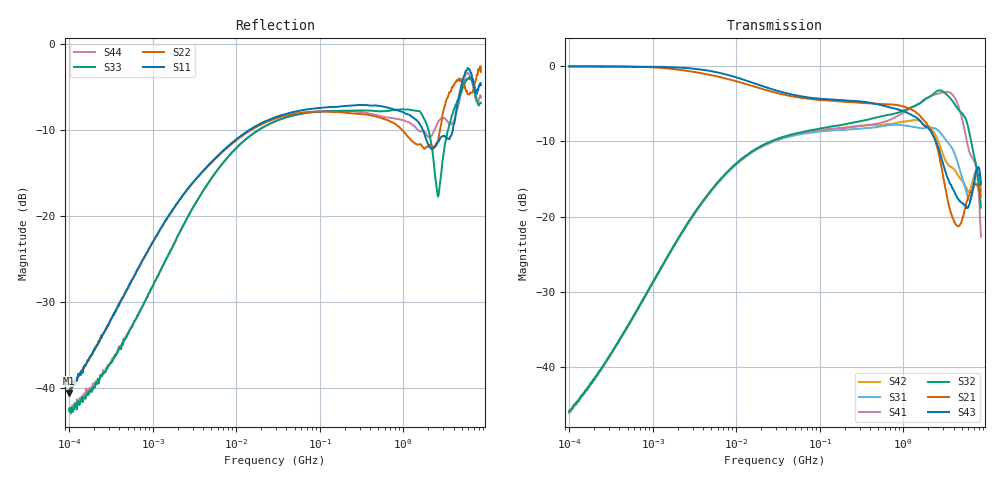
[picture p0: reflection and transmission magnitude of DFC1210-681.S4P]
# Hz S dB R 50
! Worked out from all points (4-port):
!   801 points, 100 kHz to 8.5 GHz, reference 50 ohm
!   strongest paths, dB at 100 kHz, 1.721 MHz, 29.51 MHz, 502.3 MHz, 8.5 GHz:
!     S43: -0.1, -0.2, -3.2, -5.1, -15.7
!     S21: -0.1, -0.4, -3.6, -5.1, -17.3
!     S32: -45.8, -24.2, -9.8, -6.8, -18.8
!     S41: -46.0, -24.2, -9.8, -7.6, -22.7
!     S31: -46.1, -24.3, -9.9, -8.1, -15.5
!     S42: -46.1, -24.3, -9.9, -7.8, -16.6
!   lowest |S11| = -40.6 dB at 100 kHz (marker M1), VSWR 1.02, Z = 50.4 + j0.849 ohm
!   |S11| at or under -10 dB: start of sweep to 14.49 MHz; 1.712 GHz to 3.925 GHz (2.213 GHz wide, 78.5 % of centre)
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100000  -40.61 64.6  -0.06 -0.5  -45.91 -108.0  -45.84 71.2
        -0.06 -0.5  -40.37 65.8  -45.93 72.3  -45.96 -108.8
        -46.10 -108.9  -45.84 70.8  -42.63 41.5  -0.10 -0.3
        -46.02 70.6  -46.06 -108.1  -0.10 -0.3  -42.67 49.8
2.459055e7  -8.84 21.7  -3.33 -11.9  -10.28 -154.8  -10.16 27.0
            -3.33 -11.9  -8.99 20.6  -10.13 27.6  -10.29 -154.2
            -10.29 -154.7  -10.15 27.6  -9.36 25.9  -2.97 -13.2
            -10.18 27.0  -10.30 -154.3  -2.98 -13.2  -9.36 26.0
1.357611e9  -8.68 -11.6  -6.01 -50.2  -8.13 122.0  -5.34 13.5
            -6.00 -50.2  -11.53 -15.8  -5.37 10.6  -7.21 122.7
            -8.13 121.9  -5.37 10.5  -7.76 -9.1  -6.73 -49.9
            -5.36 13.5  -7.21 122.6  -6.73 -49.9  -9.57 -8.7
2.609641e9  -11.44 65.1  -11.29 -105.3  -8.57 71.8  -3.71 -0.8
            -11.27 -105.4  -11.21 -0.0  -3.29 -2.8  -9.92 63.8
            -8.56 71.8  -3.29 -2.8  -17.78 50.5  -10.78 -99.0
            -3.71 -0.7  -9.95 63.6  -10.77 -99.0  -9.09 44.4
3.562673e9  -11.11 59.4  -18.87 -133.3  -10.48 40.4  -3.53 -17.0
            -18.81 -133.9  -5.65 29.3  -4.20 -19.9  -13.24 48.7
            -10.44 40.5  -4.20 -19.9  -9.34 76.1  -15.42 -137.7
            -3.52 -17.0  -13.29 48.5  -15.45 -137.7  -9.30 50.3
6.531769e9  -3.40 51.1  -16.63 98.4  -17.55 14.1  -11.92 -51.1
            -16.61 97.6  -5.69 20.5  -10.08 -60.1  -15.83 23.6
            -17.27 13.2  -10.08 -60.9  -4.23 44.7  -17.30 98.9
            -11.99 -51.3  -15.91 23.7  -17.41 100.1  -4.12 38.0
8.5e9  -4.79 -10.3  -17.27 47.8  -15.71 -68.4  -22.61 -110.4
       -17.31 46.7  -3.26 23.1  -18.53 -105.3  -16.32 -50.2
       -15.51 -70.6  -18.81 -106.2  -6.87 -11.4  -15.93 25.0
       -22.68 -107.5  -16.59 -49.8  -15.72 27.3  -6.27 -13.1
